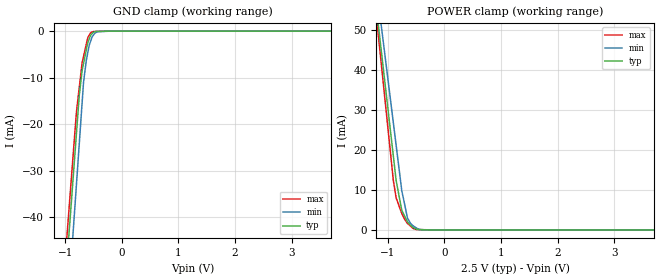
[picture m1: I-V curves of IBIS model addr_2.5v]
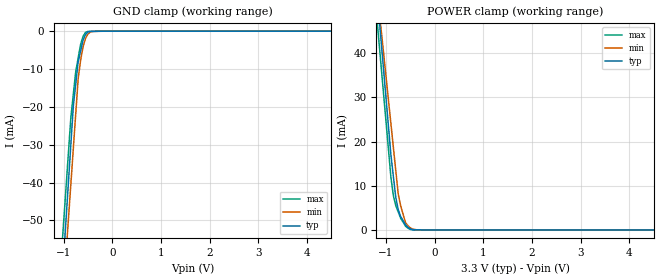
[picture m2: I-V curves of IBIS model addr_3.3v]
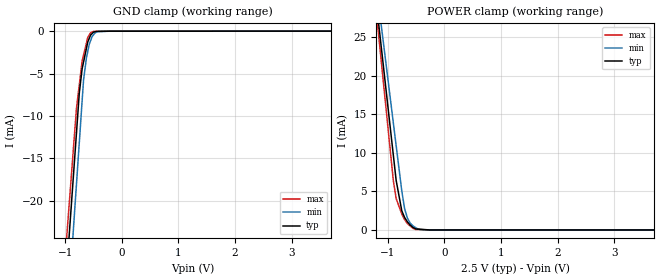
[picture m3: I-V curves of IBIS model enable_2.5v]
| Teraspeed (R) Labs.
| http://www.teraspeedlabs.com
[IBIS Ver]   3.2
[Comment Char] |_char
[File Name]   512kx32sram.ibs
[File Rev]   3.2
[Source]  Teraspeed (R) Labs.
[Date]   08-31-2016
[Notes]   Quality Check of this IBIS model: Model Passes IBIS Check
   Model parses into ICX IS. Simulation done with Hyperlynx.
   1. MIN TYP MAX information is based on Temperature and Voltage
   characteristics only.
[Disclaimer]
| Use: Teraspeed (R) Labs has licensed Teraspeed (R) AccuModel (tm)
| IBIS models to specific integrated circuit suppliers ("IC Vendors")
| for use and distribution as  follows: Each IC Vendor may use IBIS
| Models, and distribute them to IC Vendor's customers to use solely
| for developing printed circuit board designs. Users of this model may
| modify the IBIS model to suit its specific applications but
| rights to derivative works and such modifications shall belong
| to Teraspeed (R) Labs. No other distribution of these materials is
| permitted.
| DISCLAIMER OF WARRANTY: UNLESS OTHERWISE AGREED TO IN WRITING
| TERASPEED (R) LABS DISCLAIMS AND USER WAIVES ALL WARRANTIES,
| EXPRESS OR IMPLIED, INCLUDING WARRANTIES OF MERCHANTABILITY AND
| FITNESS FOR A PARTICULAR PURPOSE. IN NO EVENT SHALL
| TERASPEED BE LIABLE FOR ANY DIRECT OR INDIRECT DAMAGES,
| WHETHER IN CONTRACT OR TORT, INCLUDING, WITHOUT LIMITATION,
| LOST PROFITS, BUSINESS INTERRUPTION, OR LOST INFORMATION
| ARISING OUT OF THE USE OF OR THE INABILITY TO USE THE MODEL,
| EVEN IF TERASPEED (R) Labs HAS BEEN ADVISED OF THE POSSIBILITY
| OF SUCH DAMAGES.
[Copyright]
| This file is the legal property of Teraspeed (R) Labs Copyright(c) 2016.
| All other rights are reserved.
[Component]   512x32SRAM
[Manufacturer] Aeroflex
| 127 pin die
[Package]
| variable   typ   min   max
R_pkg  0.000E-00  0.000E-00   0.000E-00
L_pkg  0.000E-00  0.000E-00   0.000E-00
C_pkg  0.000E-00  0.000E-00   0.000E-00
[Pin] signal_name  model_name  R_pin  L_pin C_pin
1   DQ0   dq_io
2   DQ1   dq_io
3   VDDIO   POWER
4   VSS   GND
5   DQ2   dq_io
6   DQ3   dq_io
7   DQ4   dq_io
8   DQ5   dq_io
9   VSS   GND
10   VDDIO   POWER
11   DQ6   dq_io
12   DQ7   dq_io
13   VDDC   POWER
14   VDDC   POWER
15   VDDIO   POWER
16   VDDIO   POWER
17   VSS   GND
18   VSS   GND
19   VSS   GND
20   DQ8   dq_io
21   DQ9   dq_io
22   VDDIO   POWER
23   VSS   GND
24   DQ10   dq_io
25   DQ11   dq_io
26   DQ12   dq_io
27   DQ13   dq_io
28   VSS   GND
29   VDDIO   POWER
30   DQ14   dq_io
31   DQ15   dq_io
32   NC   NC
33   NC   NC
34   VDDC   POWER
35   VSS   GND
36   VSS   GND
37   VSS   GND
38   VDDC   POWER
39   VSS   GND
40   A11   addr_in
41   A12   addr_in
42   A13   addr_in
43   A14   addr_in
44   VSS   GND
45   VSS   GND
46   VDDC   POWER
47   VDDC   POWER
48   A15   addr_in
49   A16   addr_in
50   E#   en_in
51   G#   addr_in
52   VDDIO   POWER
53   SCRUB#  dq_io
54   BUSY   tri
55   MBE   dq_io
56   VSS   GND
57   VDDC   POWER
58   NC   NC
59   VSS   GND
60   NC   NC
61   VSS   GND
62   VSS   GND
63   NC   NC
64   VSS   GND
65   DQ31   dq_io
66   DQ30   dq_io
67   VDDIO   POWER
68   VSS   GND
69   DQ29   dq_io
70   DQ28   dq_io
71   DQ27   dq_io
72   DQ26   dq_io
73   VSS   GND
74   VDDIO   POWER
75   DQ25   dq_io
76   DQ24   dq_io
77   VSS   GND
78   VSS   GND
79   VDDIO   POWER
80   VDDIO   POWER
81   VDDC   POWER
82   VDDC   POWER
83   DQ23   dq_io
84   DQ22   dq_io
85   VDDIO   POWER
86   VSS   GND
87   DQ21   dq_io
88   DQ20   dq_io
89   DQ19   dq_io
90   DQ18   dq_io
91   VSS   GND
92   VDDIO   POWER
93   DQ17   dq_io
94   DQ16   dq_io
95   NC   NC
96   NC   NC
97   VSS   GND
98   VSS   GND
99   VDDIO   POWER
100   VSS   GND
101   VSS   GND
102   A10   addr_in
103   A9   addr_in
104   A8   addr_in
105   A7   addr_in
106   A6   addr_in
107   WB   addr_in
108   VSS   GND
109   VSS   GND
110   VDDC   POWER
111   VDDC   POWER
112   A18   addr_in
113   A17   addr_in
114   A5   addr_in
115   VDDIO   POWER
116   VDDIO   POWER
117   A4   addr_in
118   A3   addr_in
119   A2   addr_in
120   A1   addr_in
121   A0   addr_in
122   VSS   GND
123   VSS   GND
124   VSS   GND
125   VDDC   POWER
126   NC   NC
127   NC   NC
[Model selector] addr_in
addr_2.5v   address/ctrl input, VDD=2.5v
addr_3.3v   address/ctrl input, VDD=3.3v
[Model selector] en_in
enable_2.5v  enable input, VDD=2.5v
enable_3.3v  enable input, VDD=3.3v
[Model selector] dq_io
io_2.5v   bidir data pin, VDD=2.5v
io_3.3v   bidir data pin, VDD=3.3v
[Model selector] tri
tri_2.5v   3-state  pin, VDD=2.5v
tri_3.3v   3-state  pin, VDD=3.3v
| Models and submodels in the file (8): addr_2.5v (Input), addr_3.3v (Input), enable_2.5v (Input), enable_3.3v (Input), io_2.5v (I/O), io_3.3v (I/O), tri_2.5v (3-state), tri_3.3v (3-state)
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[Model] addr_2.5v
Model_type Input
Vinl = 800.000mV
Vinh = 2.20000V
C_comp 1.63000pF 1.62000pF 1.64000pF
| variable typ   min   max
[Voltage Range] 2.50000V 2.30000V 2.70000V
[POWER Clamp Reference] 2.50000V 2.30000V 2.70000V
[GND Clamp Reference] 0.00000V 0.00000V 0.00000V
[Temperature Range]   25   105   -55
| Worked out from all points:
|   GND clamp passes 1 mA (typ) near -0.55 V on its own axis
|   POWER clamp passes 1 mA (typ) near -0.58 V on its own axis
[GND Clamp]
-2.5V     -299.9mA   -330.6mA   -287.2mA
-800mV    -21.9mA    -32.84mA   -17.3mA
-750mV    -13.73mA   -24.08mA   -12.03mA
-700mV    -8.464mA   -15.32mA   -6.76mA
-675mV    -6.956mA   -10.94mA   -5.417mA
-625mV    -3.938mA   -6.162mA   -2.732mA
-600mV    -2.429mA   -4.599mA   -1.389mA
-575mV    -1.656mA   -3.035mA   -868.2uA
-500mV    -228.2uA   -843.3uA   -56.41uA
-425mV    -38.52uA   -107.2uA   -40.1uA
-212.5mV  -2.335uA   -2.292uA   -1.978uA
5V        8.86uA     20.32uA    7.649uA
[POWER Clamp]
-2.5V     216mA      208.7mA    231.3mA
-1.1V     43.21mA    49.56mA    39.79mA
-900mV    18.52mA    26.83mA    12.43mA
-850mV    12.35mA    21.15mA    8.018mA
-750mV    4.879mA    9.782mA    4.104mA
-700mV    3.471mA    6.391mA    2.656mA
-650mV    2.063mA    2.999mA    1.633mA
-600mV    1.239mA    1.721mA    1.012mA
-550mV    640uA      1.027mA    390.3uA
-425mV    64.8uA     118.4uA    85.46uA
-275mV    16.2uA     0A         38.85uA
5V        0A         0A         0A
[Model] addr_3.3v
Model_type Input
Vinl = 800.000mV
Vinh = 2.20000V
C_comp 3.63000pF 3.62000pF 3.64000pF
| variable typ   min   max
[Voltage Range] 3.30000V 3.00000V 3.60000V
[POWER Clamp Reference] 3.30000V 3.00000V 3.60000V
[GND Clamp Reference] 0.00000V 0.00000V 0.00000V
[Temperature Range]   25   105   -55
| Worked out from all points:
|   GND clamp passes 1 mA (typ) near -0.55 V on its own axis
|   POWER clamp passes 1 mA (typ) near -0.58 V on its own axis
[GND Clamp]
-3.3V     -522.2mA   -494.6mA   -480mA
-850mV    -29.9mA    -40.4mA    -22.76mA
-800mV    -19.85mA   -31.13mA   -16.74mA
-750mV    -13.97mA   -21.86mA   -10.71mA
-700mV    -8.091mA   -12.59mA   -7.104mA
-650mV    -5.233mA   -7.693mA   -3.5mA
-600mV    -2.375mA   -4.148mA   -1.355mA
-550mV    -872.6uA   -1.951mA   -340.6uA
-500mV    -227.2uA   -748.5uA   -55.24uA
-400mV    -34.15uA   -51.98uA   -34.01uA
-200mV    -2.575uA   -3.043uA   -2.105uA
6.6V      9.583uA    36.64uA    4.888uA
[POWER Clamp]
-3.3V     323.9mA    278.3mA    311.4mA
-1.2V     55.29mA    55.78mA    49.32mA
-1.15V    48.89mA    50.48mA    43.08mA
-1.1V     42.5mA     45.18mA    36.84mA
-900mV    16.91mA    23.99mA    11.88mA
-850mV    12.13mA    18.69mA    7.773mA
-800mV    7.338mA    13.39mA    5.502mA
-750mV    4.605mA    8.093mA    4.081mA
-700mV    3.057mA    5.464mA    2.66mA
-600mV    1.182mA    1.666mA    868.3uA
-500mV    236.2uA    472.7uA    115uA
6.6V      0A         0A         0A
[Model] enable_2.5v
Model_type Input
Vinl = 800.000mV
Vinh = 2.20000V
C_comp 1.50000pF 1.44000pF 1.56000pF
| variable typ   min   max
[Voltage Range] 2.50000V 2.30000V 2.70000V
[POWER Clamp Reference] 2.50000V 2.30000V 2.70000V
[GND Clamp Reference] 0.00000V 0.00000V 0.00000V
[Temperature Range]   25   105   -55
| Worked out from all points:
|   GND clamp passes 1 mA (typ) near -0.58 V on its own axis
|   POWER clamp passes 1 mA (typ) near -0.65 V on its own axis
[GND Clamp]
-2.5V     -171.8mA   -184.9mA   -158.7mA
-800mV    -11.99mA   -18.03mA   -9.093mA
-750mV    -7.287mA   -13.12mA   -6.302mA
-700mV    -4.43mA    -8.215mA   -3.512mA
-675mV    -3.637mA   -5.761mA   -2.814mA
-625mV    -2.051mA   -3.195mA   -1.417mA
-600mV    -1.257mA   -2.38mA    -719.1uA
-575mV    -857.1uA   -1.566mA   -450.1uA
-550mV    -456.8uA   -1.11mA    -181.1uA
-475mV    -70.92uA   -218.2uA   -27.15uA
-212.5mV  -2.105uA   -1.913uA   -1.988uA
5V        6.77uA     12.39uA    6.023uA
[POWER Clamp]
-2.5V     115mA      108.7mA    122.7mA
-1.1V     22.89mA    25.77mA    20.96mA
-900mV    9.729mA    13.92mA    6.424mA
-850mV    6.44mA     10.96mA    4.081mA
-750mV    2.478mA    5.038mA    2.067mA
-700mV    1.612mA    2.747mA    1.334mA
-650mV    1.039mA    1.518mA    819.6uA
-600mV    623.7uA    866.7uA    507.4uA
-550mV    321.1uA    517.4uA    195.3uA
-425mV    89.72uA    59.96uA    43.18uA
-275mV    12.82uA    0A         19.63uA
5V        0A         0A         0A
